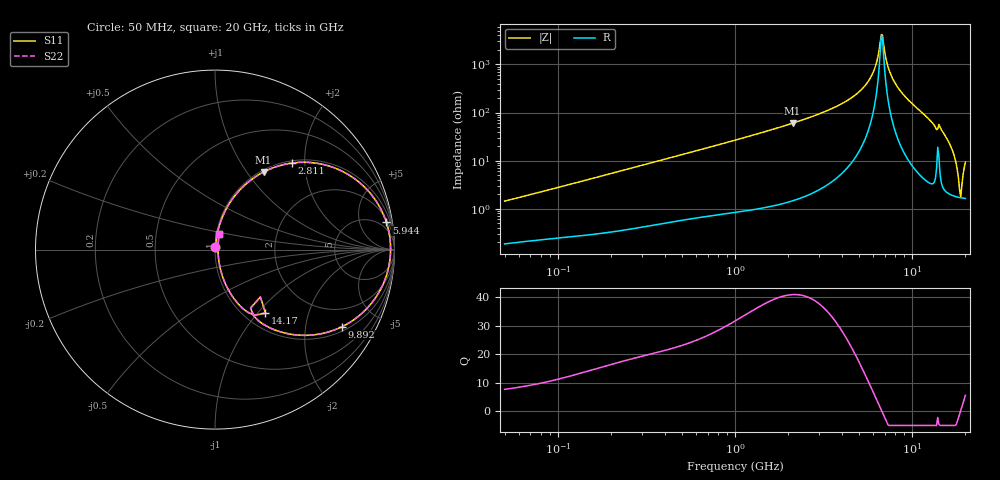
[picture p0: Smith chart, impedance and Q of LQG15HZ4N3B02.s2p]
!Murata Part Number: LQG15HZ4N3B02
!These Parameters are Measured in Series Mode Connection
!  o--[Z]--o
!Port1  Port2
!  o-------o
!Freq. Start=50[MHz] Stop=20[GHz], 401[Steps]
# Hz S RI R 50
!Freq.(Hz) S11(Real) S11(Imag) S21(Real) S21(Imag) S12(Real) S12(Imag) S22(Real) S22(Imag)
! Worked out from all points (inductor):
!   401 points, 50 MHz to 20 GHz, reference 50 ohm
!   read as one part in series: L = 4.49 nH near 51.52 MHz
!   highest Q = 41 at 2.115 GHz (marker M1), where L = 4.52 nH
!   self-resonance near 6.701 GHz
!   S11 on the Smith chart (normalised r, x): 50 MHz: 1.00, +0.03; 2.811 GHz: 1.04, +1.72; 5.944 GHz: 3, +12; 9.892 GHz: 1.17, -3.19; 14.17 GHz: 1.24, -1.10; 20 GHz: 1.03, +0.18
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5e7  0.00206 0.0143  0.9979 -0.0143  0.9979 -0.0143  0.00206 0.0143
1.364002e8  0.00414 0.0371  0.9959 -0.0371  0.9959 -0.0371  0.00414 0.0371
3.721004e8  0.0144 0.0977  0.9856 -0.0977  0.9856 -0.0977  0.0144 0.0977
1e9  0.073 0.2449  0.927 -0.2449  0.927 -0.2449  0.073 0.2449
2.114743e9  0.2703 0.4321  0.7297 -0.4321  0.7297 -0.4321  0.2703 0.4321
2.728004e9  0.4089 0.4791  0.5911 -0.4791  0.5911 -0.4791  0.4089 0.4791
2.810964e9  0.4282 0.4821  0.5718 -0.4821  0.5718 -0.4821  0.4282 0.4821
4.539627e9  0.7929 0.3836  0.2071 -0.3836  0.2071 -0.3836  0.7929 0.3836
5.352748e9  0.9055 0.2582  0.0945 -0.2582  0.0945 -0.2582  0.9055 0.2582
5.944466e9  0.9551 0.1512  0.0449 -0.1512  0.0449 -0.1512  0.9551 0.1512
6.701223e9  0.9783 0.00862  0.0217 -0.00862  0.0217 -0.00862  0.9783 0.00862
6.905011e9  0.9773 -0.0293  0.0227 0.0293  0.0227 0.0293  0.9773 -0.0293
7.442007e9  0.9609 -0.1254  0.0391 0.1254  0.0391 0.1254  0.9609 -0.1254
8.264682e9  0.9026 -0.2561  0.0974 0.2561  0.0974 0.2561  0.9026 -0.2561
9.892087e9  0.7085 -0.4291  0.2915 0.4291  0.2915 0.4291  0.7085 -0.4291
1.201863e10  0.41 -0.4693  0.59 0.4693  0.59 0.4693  0.41 -0.4693
1.417136e10  0.2813 -0.3535  0.7187 0.3535  0.7187 0.3535  0.2813 -0.3535
1.670968e10  0.0487 -0.1683  0.9513 0.1683  0.9513 0.1683  0.0487 -0.1683
1.747767e10  0.0288 -0.1033  0.9712 0.1033  0.9712 0.1033  0.0288 -0.1033
1.855685e10  0.0171 -0.0165  0.9829 0.0165  0.9829 0.0165  0.0171 -0.0165
1.912117e10  0.0172 0.0261  0.9828 -0.0261  0.9828 -0.0261  0.0172 0.0261
2e10  0.0241 0.088  0.9759 -0.088  0.9759 -0.088  0.0241 0.088
